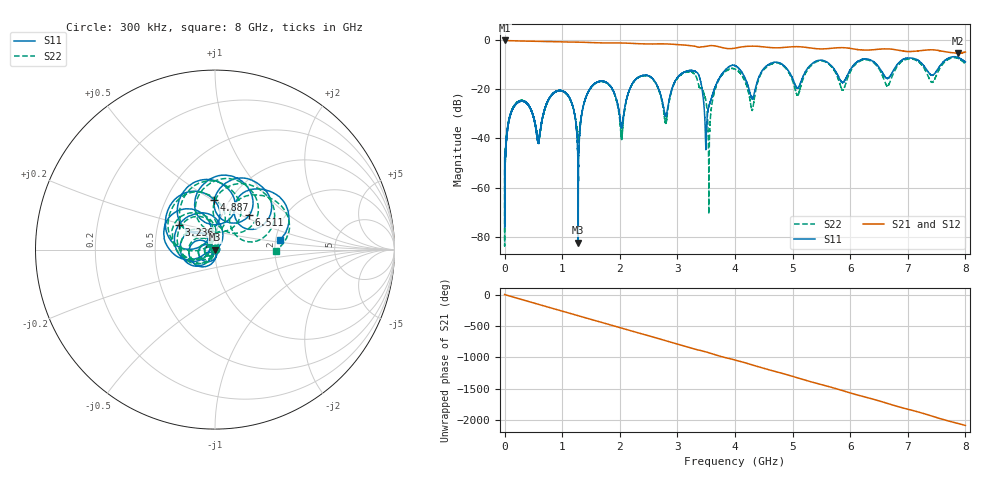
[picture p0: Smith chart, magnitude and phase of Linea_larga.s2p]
#  HZ  S  DB  R  50.00
! Rohde & Schwarz ZVA/B
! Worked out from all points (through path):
!   30000 points, 300 kHz to 8 GHz, reference 50 ohm
!   highest |S21| = 0.00 dB at 566.7 kHz (marker M1); lowest = -5.2 dB at 7.878 GHz (marker M2)
!   group delay of S21, straight-line fit = 723 ps
!   lowest |S11| = -82.5 dB at 1.279 GHz (marker M3), VSWR 1.00, Z = 50 - j0.00656 ohm
!   |S11| at or under -10 dB: start of sweep to 4.572 GHz; 4.834 GHz to 5.312 GHz (478.1 MHz wide, 9.42 % of centre); 5.661 GHz to 6.061 GHz (400.5 MHz wide, 6.83 % of centre)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
!   |S22| runs from -83.9 to -7.0 dB; largest |S21 - S12| = 0.0064
!   S11 on the Smith chart (normalised r, x): 300 kHz: 1.00, +0.01; 3.236 GHz: 0.64, +0.19; 4.887 GHz: 0.85, +0.51; 6.511 GHz: 1.34, +0.56; 8 GHz: 2.10, +0.26
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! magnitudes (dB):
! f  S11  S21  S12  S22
! 300 kHz  -47.8  0.0  0.0  -52.7
! 566.7 kHz  -58.2  0.0  0.0  -63.9
! 183.8 MHz  -26.2  -0.2  -0.2  -26.2
! 585.9 MHz  -41.2  -0.4  -0.4  -40.3
! 937.6 MHz  -20.5  -0.6  -0.6  -20.5
! 1.279 GHz  -82.5  -0.7  -0.7  -41.1
! 1.334 GHz  -30.7  -0.7  -0.7  -31.0
! 1.615 GHz  -16.9  -0.9  -1.0  -17.0
! 2.03 GHz  -35.4  -1.0  -1.0  -39.8
! 2.269 GHz  -16.0  -1.3  -1.3  -16.1
! 2.667 GHz  -19.4  -1.4  -1.4  -19.7
! 2.799 GHz  -30.7  -1.4  -1.4  -33.8
! 3.236 GHz  -12.3  -2.1  -2.1  -12.8
! 3.551 GHz  -26.6  -2.1  -2.2  -47.5
! 4 GHz  -10.3  -3.1  -3.1  -11.7
! 4.296 GHz  -23.6  -2.3  -2.3  -28.3
! 4.887 GHz  -11.2  -2.8  -2.8  -11.6
! 5.334 GHz  -9.5  -3.1  -3.1  -10.0
! 6.511 GHz  -11.4  -3.5  -3.5  -12.0
! 6.667 GHz  -15.3  -3.4  -3.4  -18.1
! 7.878 GHz  -7.0  -5.2  -5.2  -7.4
! 8 GHz  -8.8  -4.7  -4.8  -9.5
